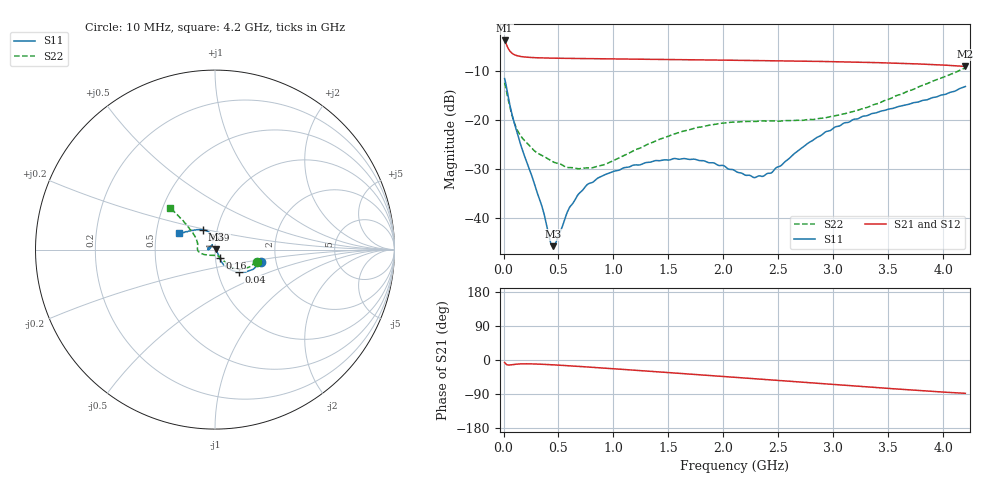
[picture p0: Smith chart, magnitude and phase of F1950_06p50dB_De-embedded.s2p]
! Integrated Device Technology
! Corporate Headquarters
! 6024 Silver Creek Valley Road
! San Jose, CA 95138  USA
! Phone:  1-408-284-8200
! Toll Free:  1-800-223-1366
! Webpage:  http://www.idt.com/
! Timing and RF Division
! 515 Groton Road, Suite 102
! Westford, MA 01886-6024
! Device:  F1950
! Description: 7-bit 0.25 dB Digital Step Attenuator
! Frequency:  150.0 -  4000.00 MHz
! Package:  4x4 mm Thin QFN Plastic Package: 24 pin
! Ports:  2 RF, 12 DC
!  Pin  1  = D0
!  Pin  2  = VDD
!  Pin  3  = Vmode
!  Pin  4  = GND
!  Pin  5  = RF1  =  Port 1
!  Pin  6  = GND
!  Pin  7  = GND
!  Pin  8  = GND
!  Pin  9  = GND
!  Pin 10  = GND
!  Pin 11  = GND
!  Pin 12  = GND
!  Pin 13  = GND
!  Pin 14  = RF2  =  Port 2
!  Pin 15  = GND
!  Pin 16  = LE
!  Pin 17  = CLK
!  Pin 18  = DATE
!  Pin 19  = D6
!  Pin 20  = D5
!  Pin 21  = D4
!  Pin 22  = D3
!  Pin 23  = D2
!  Pin 24  = D1
! State:  26
! Atten State:  6.50 dB
! Voltage:  +5.00 Volts
! Current:  Not Measured mA
! Data:  The device was measured on a the F195X evaluation board which has
!  individual transmission lines to the RF pins.  Data was collected
!  using a calibrated network analyzer.  The evaluation board was
!  de-embedded using a TRL calibration technique.
!  The reference plane is the edge of the package pin.
! Misc:  Board 2019
!  Action Tracker AT0250
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# GHz S dB R 50
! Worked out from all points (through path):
!   420 points, 10 MHz to 4.2 GHz, reference 50 ohm
!   highest |S21| = -3.73 dB at 10 MHz (marker M1); lowest = -9.0 dB at 4.2 GHz (marker M2)
!   group delay of S21, straight-line fit = 55.6 ps
!   lowest |S11| = -45.6 dB at 450 MHz (marker M3), VSWR 1.01, Z = 50.5 + j0.216 ohm
!   |S11| at or under -10 dB: start of sweep to end of sweep
!   |S22| runs from -29.9 to -9.3 dB; largest |S21 - S12| = 0.00055
!   S11 on the Smith chart (normalised r, x): 10 MHz: 1.67, -0.24; 40 MHz: 1.26, -0.33; 160 MHz: 1.05, -0.10; 3.49 GHz: 0.86, +0.19; 4.2 GHz: 0.66, +0.13
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0.01  -11.50 -14.5  -3.73 -6.6  -3.72 -6.6  -12.33 -16.0
0.04  -14.80 -43.4  -5.23 -13.1  -5.23 -13.1  -15.47 -40.8
0.1  -20.70 -60.9  -6.64 -11.5  -6.64 -11.5  -20.62 -51.2
0.16  -25.25 -62.0  -7.01 -10.3  -7.00 -10.3  -23.27 -54.5
0.34  -36.89 -43.1  -7.28 -11.1  -7.28 -11.1  -27.04 -61.4
0.42  -44.21 -7.4  -7.32 -12.3  -7.32 -12.3  -28.04 -64.2
0.45  -45.65 24.2  -7.33 -12.7  -7.33 -12.7  -28.46 -67.0
0.49  -44.06 65.8  -7.35 -13.4  -7.35 -13.4  -28.75 -70.8
0.59  -38.21 104.2  -7.38 -15.2  -7.38 -15.2  -29.63 -79.2
0.71  -34.44 119.7  -7.41 -17.4  -7.41 -17.4  -29.81 -92.0
0.77  -32.96 124.2  -7.43 -18.6  -7.43 -18.6  -29.72 -98.5
0.94  -30.92 137.5  -7.47 -21.9  -7.47 -21.9  -28.82 -118.7
1.41  -28.22 167.5  -7.59 -31.4  -7.59 -31.4  -23.92 -153.8
1.74  -27.93 180.0  -7.67 -38.2  -7.67 -38.2  -21.58 -166.4
2.11  -30.35 173.3  -7.77 -45.9  -7.76 -45.9  -20.36 -177.1
2.28  -31.68 151.5  -7.81 -49.4  -7.81 -49.4  -20.23 178.5
2.37  -31.30 136.5  -7.84 -51.2  -7.84 -51.3  -20.13 176.0
2.81  -24.12 101.8  -7.97 -60.5  -7.97 -60.5  -19.84 161.2
3.1  -20.52 106.5  -8.09 -66.6  -8.08 -66.7  -18.67 152.1
3.49  -17.79 120.9  -8.30 -74.7  -8.30 -74.8  -15.79 142.5
3.51  -17.67 122.0  -8.31 -75.2  -8.31 -75.2  -15.65 142.0
4.2  -13.11 155.6  -9.02 -87.9  -9.02 -88.0  -9.32 137.1
